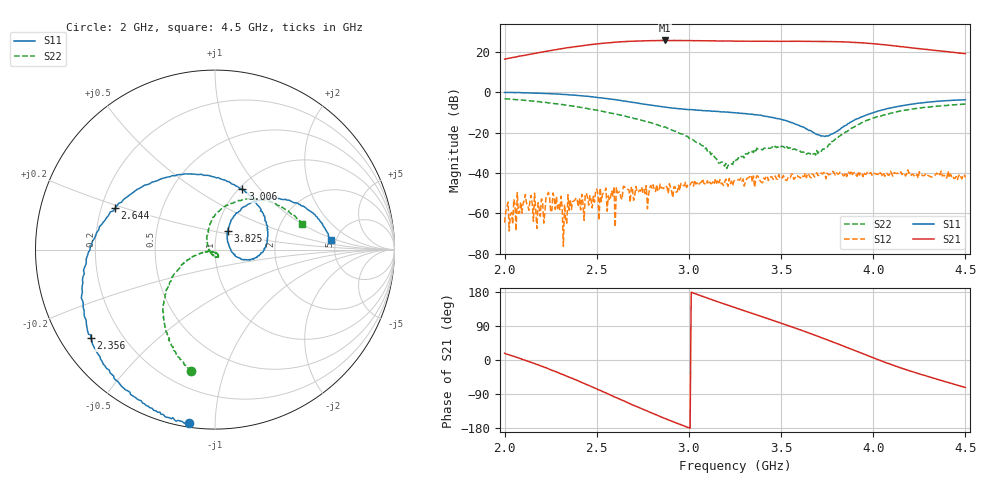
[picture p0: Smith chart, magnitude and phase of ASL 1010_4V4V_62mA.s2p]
!ASL 1010 Low Noise Amplifier
!Test-Fixture S-parameter data in 2.0- 4.5 GHz
!Bias conditions Vd1=4V,Vd2=4V, Ids =62mA
!Agilent Technologies,N5230A,MY45000233,A.04.83
!Agilent N5230A: A.04.83
!Date: Tuesday, July 25, 2006 23:01:20
!Correction: S11(Full 2 Port SOLT,1,2) S21(Full 2 Port SOLT,1,2) S12(Full 2 Port SOLT,1,2) S22(Full 2 Port SOLT,1,2)
!S2P File: Measurements: S11, S21, S12, S22:
# Hz S  dB  R 50
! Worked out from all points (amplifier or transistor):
!   401 points, 2 GHz to 4.5 GHz, reference 50 ohm
!   highest |S21| = 25.5 dB at 2.869 GHz (marker M1)
!   |S21| within 3 dB of that: 2.39 GHz to 4.143 GHz (1.753 GHz wide, 53.7 % of centre)
!   unconditionally stable (mu >= 1): 2.073 GHz to 2.108 GHz; 2.115 GHz to 2.162 GHz; 2.163 GHz to end of sweep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
!   at 2.413 GHz: K = 7.99, MAG = 28.5 dB, |S12| = -58.3 dB
!   at 3.25 GHz: K = 3.82, MAG = 25.6 dB, |S12| = -43.5 dB
!   at 4.5 GHz: K = 3.36, MAG = 22.5 dB, |S12| = -42.3 dB
!   S11 on the Smith chart (normalised r, x): 2 GHz: 0.02, -0.86; 2.356 GHz: 0.09, -0.32; 2.644 GHz: 0.26, +0.19; 3.006 GHz: 1.04, +0.81; 3.825 GHz: 1.13, +0.24; 4.5 GHz: 4.52, +0.83
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2e9  -0.19 -98.4  16.25 17.9  -64.56 77.5  -3.24 -101.0
2.16875e9  -0.55 -117.1  19.20 -10.9  -58.08 -109.3  -4.63 -114.3
2.28125e9  -0.95 -132.3  21.00 -31.4  -51.55 125.6  -5.79 -123.1
2.35625e9  -1.40 -144.6  22.09 -46.7  -53.05 113.6  -6.76 -129.4
2.41875e9  -1.89 -155.0  22.87 -59.2  -50.55 -162.2  -7.70 -133.4
2.5375e9  -3.02 -178.7  24.15 -84.5  -49.74 171.1  -9.61 -142.2
2.64375e9  -4.40 157.6  24.90 -107.4  -46.64 158.6  -11.67 -149.5
2.73125e9  -5.63 136.2  25.22 -126.0  -48.53 144.0  -13.71 -155.6
2.8375e9  -7.04 108.4  25.44 -147.9  -48.74 104.9  -16.47 -159.7
2.86875e9  -7.41 100.2  25.49 -154.1  -46.64 110.3  -17.17 -161.6
3.00625e9  -8.63 65.6  25.39 -180.0  -45.91 84.5  -23.00 -167.2
3.1e9  -9.29 45.3  25.33 163.5  -43.80 90.2  -29.18 -161.4
3.25e9  -10.25 17.0  25.15 138.2  -43.54 60.2  -34.31 -68.8
3.35625e9  -11.26 1.2  25.09 120.9  -47.12 43.0  -28.20 -63.7
3.475e9  -12.99 -12.9  25.09 101.4  -42.94 43.1  -27.43 -74.0
3.58125e9  -16.00 -20.5  25.07 83.5  -41.19 5.3  -28.58 -98.1
3.66875e9  -19.59 -12.1  25.05 68.1  -40.55 -11.2  -31.10 -153.6
3.825e9  -17.93 55.3  24.81 39.2  -39.67 -25.1  -21.19 122.2
3.95e9  -11.85 57.2  24.24 15.2  -39.65 -37.4  -14.72 91.2
4.0875e9  -8.02 45.7  23.07 -10.3  -40.94 -82.8  -10.64 65.7
4.26875e9  -5.29 26.5  21.23 -39.4  -41.31 -92.5  -7.66 39.6
4.5e9  -3.77 4.7  19.02 -72.5  -42.30 -143.3  -5.91 16.7
